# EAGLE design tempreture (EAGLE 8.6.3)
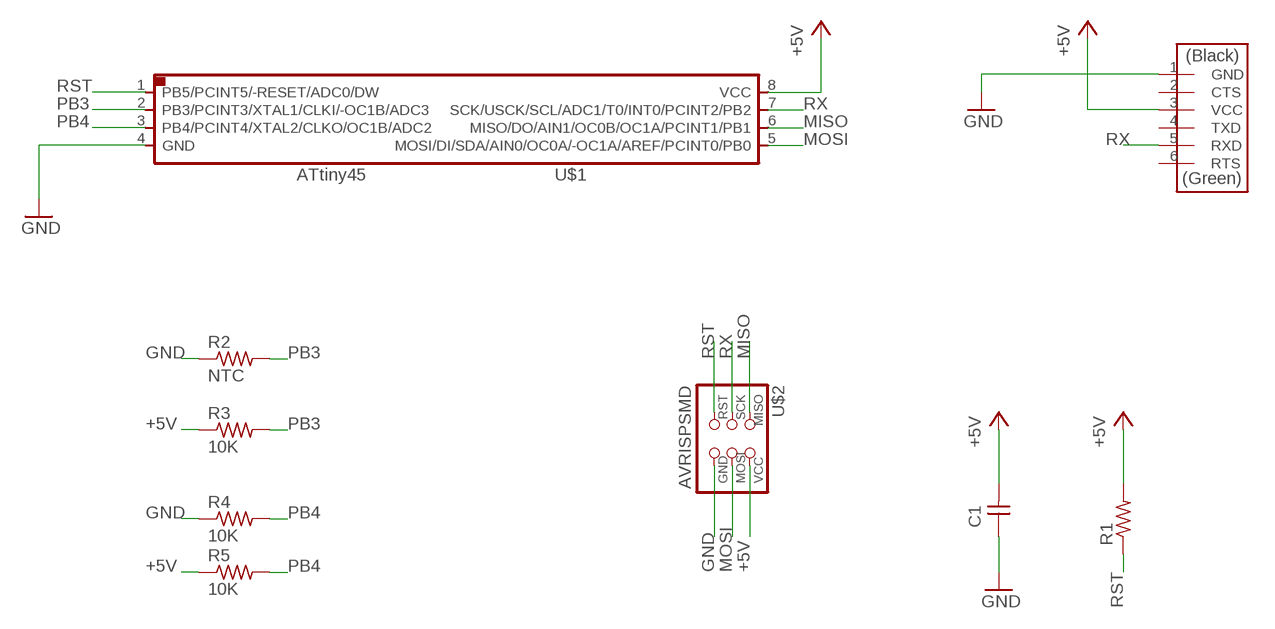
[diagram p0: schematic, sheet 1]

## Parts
C1  CAP-UNPOLARIZEDFAB  [C1206FAB]
R1  RES-US1206FAB  [R1206FAB]
R2  NTC  RES-US1206FAB  [R1206FAB]
R3  10K  RES-US1206FAB  [R1206FAB]
R4  10K  RES-US1206FAB  [R1206FAB]
R5  10K  RES-US1206FAB  [R1206FAB]
U$1  ATTINY45SI  [SOIC8]
U$2  AVRISPSMD  [2X03SMD]
U$3  FTDI-SMD-HEADER  [1X06SMD]

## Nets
+5V: C1.2 R1.2 R3.1 R5.1 U$1.8(VCC) U$2.2(VCC) U$3.3(VCC)
GND: C1.1 R2.1 R4.1 U$1.4(GND) U$2.6(GND) U$3.1(GND)
MISO: U$1.6(MISO/DO/AIN1/OC0B/OC1A/PCINT1/PB1) U$2.1(MISO)
MOSI: U$1.5(MOSI/DI/SDA/AIN0/OC0A/-OC1A/AREF/PCINT0/PB0) U$2.4(MOSI)
PB3: R2.2 R3.2 U$1.2(PB3/PCINT3/XTAL1/CLKI/-OC1B/ADC3)
PB4: R4.2 R5.2 U$1.3(PB4/PCINT4/XTAL2/CLKO/OC1B/ADC2)
RST: R1.1 U$1.1(PB5/PCINT5/-RESET/ADC0/DW) U$2.5(RST)
RX: U$1.7(SCK/USCK/SCL/ADC1/T0/INT0/PCINT2/PB2) U$2.3(SCK) U$3.5(RXD)
Unconnected: U$3.2(CTS) U$3.4(TXD) U$3.6(RTS)

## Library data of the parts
C1 = fab:CAP-UNPOLARIZED
R1 = fab:RES-US: Resistor (US Symbol)
R2-R5 = HelloKamakura:RES-US: Resistor (US Symbol)
U$1 = fab:ATTINY45
U$2 = fab:AVRISP
U$3 = fab:FTDI-SMD-HEADER

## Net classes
0 default: width 0.406 mm

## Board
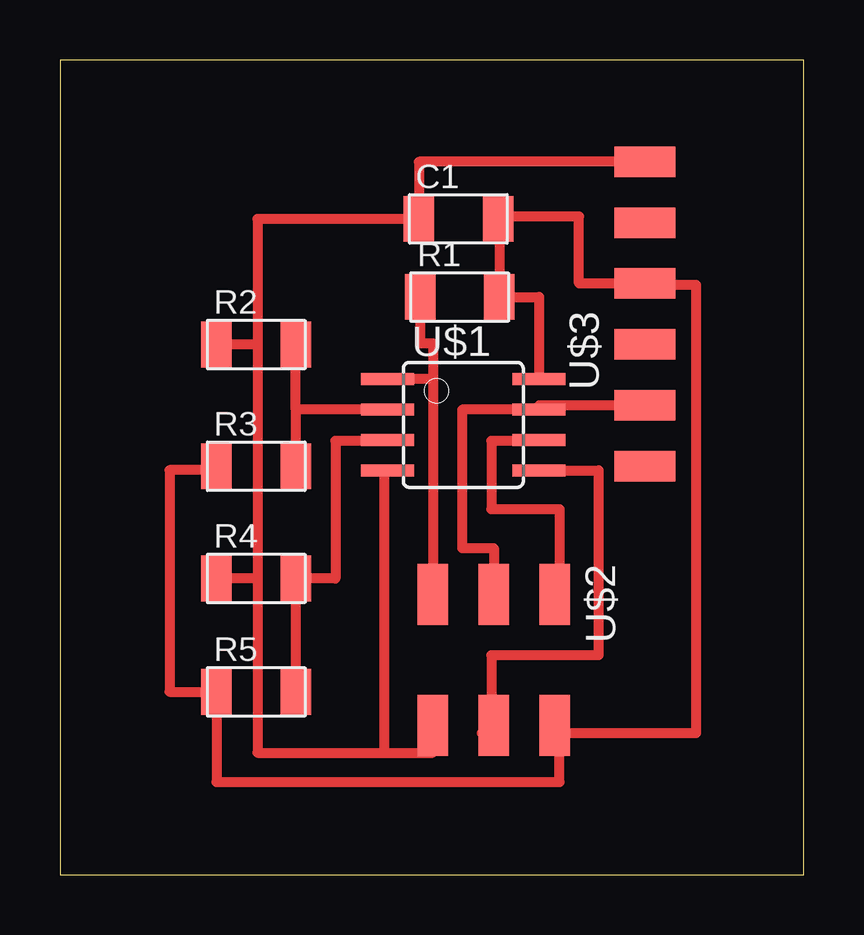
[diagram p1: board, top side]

Size 31.02 x 33.96 mm. Coordinates in mm from the lower left corner, seen from the top.
Outline: 0,0 31.02,0 31.02,33.96 0,33.96 0,0
Copper layers (1*16): Top 0.035mm / dielectric 1.5mm / Bottom 0.035mm
Design rules "default *": minimum track width 6mil, minimum drill 0.35mm, track to track 0.4mm, track to pad 0.4mm, pad to pad 0.4mm, via to via 0.4mm, smd to smd 0.4mm, copper to edge 40mil, drill to drill 6mil, minimum pad ring 10mil, minimum via ring 8mil, stop-mask expansion 4mil, vias tented up to drill 0mil, thermal gap 10mil

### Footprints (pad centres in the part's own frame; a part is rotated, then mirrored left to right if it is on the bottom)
C1206FAB = smd 1.27 x 1.905: 1 -1.651,0; 2 1.651,0
R1206FAB = smd 1.27 x 1.905: 1 -1.651,0; 2 1.651,0
SOIC8 = smd 0.5 x 2.2: 1 -1.905,-3.154; 2 -0.645,-3.154; 3 0.625,-3.154; 4 1.895,-3.154; 5 1.905,3.154; 6 0.635,3.154; 7 -0.635,3.154; 8 -1.905,3.154
2X03SMD = smd 2.54 x 1.27: 1 -2.54,2.54; 2 2.92,2.54; 3 -2.54,0; 4 2.92,0; 5 -2.54,-2.54; 6 2.92,-2.54
1X06SMD = smd 2.54 x 1.27: 1 0,6.35; 2 0,3.81; 3 0,1.27; 4 0,-1.27; 5 0,-3.81; 6 0,-6.35

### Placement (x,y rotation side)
C1  16.61,27.33 0 top
R1  16.66,24.08 0 top
R2  8.18,22.1 0 top
R3  8.18,17.02 0 top
R4  8.18,12.34 0 top
R5  8.18,7.62 0 top
U$1  16.81,18.75 270 top
U$2  18.08,9.14 270 top
U$3  24.38,23.37 0 top

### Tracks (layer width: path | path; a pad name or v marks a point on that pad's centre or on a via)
+5V
  Top 0.406: R3.1 6.53,16.87 4.57,16.87 4.57,7.62 R5.1 6.53,3.86 20.83,3.86 20.83,5.89 | U$1.8 19.97,24.08 R1.2 18.31,27.33 C1.2 18.26,27.43 21.64,27.43 21.64,24.64 U$3.3 24.38,24.59 26.52,24.59 26.52,5.89 20.83,5.89 | U$2.2 20.83,6.22 20.83,5.89
GND
  Top 0.406: U$3.1 14.96,29.72 C1.1 8.23,27.33 8.23,22.1 | 8.23,12.34 R4.1 | 8.23,22.1 8.23,12.34 | 8.23,22.1 R2.1 | 8.23,12.34 8.23,5.08 13.51,5.08 | U$2.6 15.54,5.08 13.51,5.08 | U$1.4 13.51,16.85 13.51,5.08
MISO
  Top 0.406: U$1.6 19.97,18.09 17.98,18.09 17.98,15.24 20.83,15.24 20.83,11.68 U$2.1
MOSI
  Top 0.406: U$1.5 22.45,16.84 | 22.45,16.84 22.45,16.87 | 22.45,16.84 22.45,9.14 17.98,9.14 17.98,5.89 | 17.98,5.89 17.58,5.89 | 17.98,5.89 18.09,5.89 U$2.4
PB3
  Top 0.406: U$1.2 9.83,19.39 | 9.83,19.39 R2.2 | 9.83,19.39 R3.2
PB4
  Top 0.406: R5.2 R4.2 11.48,12.34 11.48,18.09 13.66,18.09 U$1.3
RST
  Top 0.406: R1.1 15.01,22.15 15.54,22.15 15.54,20.65 | 15.54,20.65 U$2.5 | 15.54,20.65 U$1.1
RX
  Top 0.406: U$3.5 19.97,19.56 U$1.7 16.76,19.38 16.76,13.61 18.09,13.61 U$2.3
